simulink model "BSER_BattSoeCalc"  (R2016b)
settings: Solver=FixedStepDiscrete  StartTime=0.0  StopTime=10.0  FixedStep=0.02  RelTol=1e-3  EnableMultiTasking=on
undefined symbols (not defined in the file or in its folder): BSER_ahBattCapFilter_C, BSER_ahBattCapTemp_CUR, BSER_ahBattNrmCap_C, BSER_eBattSoeFilter_C, BSER_numSoeSeriesCells_C, BSER_rOCVSoc_A, BSER_rShrtPwrMapSoc_A, BSER_rSoeUsableRate_C, BSER_tBattCapTemp_A, BSER_tiSoeIniTime_C, BSER_uBattNrmVolt_C, BSER_uOCVSoc_CUR
libraries: simulink x4

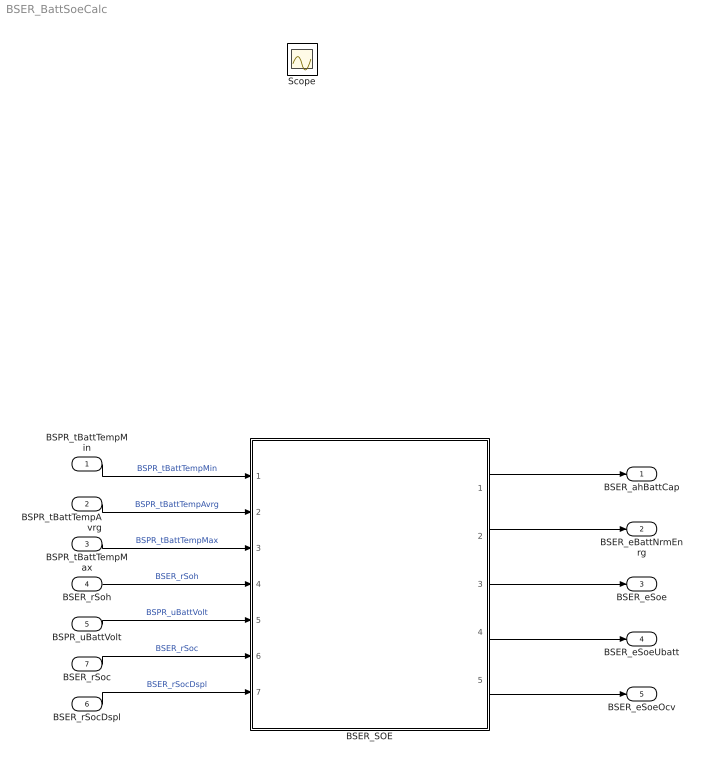
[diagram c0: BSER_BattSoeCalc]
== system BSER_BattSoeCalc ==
  BSPR_tBattTempMin : Inport
  BSPR_tBattTempAvrg : Inport  Port=2
  BSPR_tBattTempMax : Inport  Port=3
  BSER_rSoh : Inport  Port=4
  BSPR_uBattVolt : Inport  Port=5
  BSER_rSocDspl : Inport  Port=6
  BSER_rSoc : Inport  Port=7
  BSER_SOE : Subsystem  TreatAsAtomicUnit=on
  BSER_ahBattCap : Outport
  BSER_eBattNrmEnrg : Outport  Port=2
  BSER_eSoe : Outport  Port=3
  BSER_eSoeUbatt : Outport  Port=4
  BSER_eSoeOcv : Outport  Port=5
  Scope : Scope
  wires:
  BSPR_tBattTempAvrg/1 -> BSER_SOE/2(BSPR_tBattTempAvrg)  "BSPR_tBattTempAvrg"
  BSPR_tBattTempMin/1 -> BSER_SOE/1(BSPR_tBattTempMin)  "BSPR_tBattTempMin"
  BSPR_tBattTempMax/1 -> BSER_SOE/3(BSPR_tBattTempMax)  "BSPR_tBattTempMax"
  BSER_SOE/1(BSER_ahBattCap) -> BSER_ahBattCap/1
  BSER_rSoh/1 -> BSER_SOE/4(BSER_rSoh)  "BSER_rSoh"
  BSPR_uBattVolt/1 -> BSER_SOE/5(BSPR_uBattVolt)  "BSPR_uBattVolt"
  BSER_rSocDspl/1 -> BSER_SOE/7(BSER_rSocDspl)  "BSER_rSocDspl"
  BSER_SOE/2(BSER_eBattNrmEnrg) -> BSER_eBattNrmEnrg/1
  BSER_SOE/3(BSER_eSoe) -> BSER_eSoe/1
  BSER_SOE/4(BSER_eSoeUbatt) -> BSER_eSoeUbatt/1
  BSER_rSoc/1 -> BSER_SOE/6(BSER_rSoc)  "BSER_rSoc"
  BSER_SOE/5(BSER_eSoeOcv) -> BSER_eSoeOcv/1

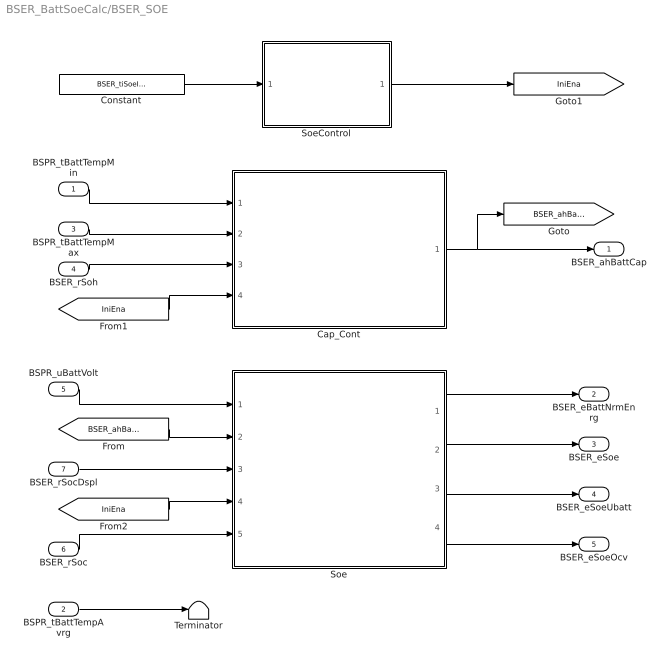
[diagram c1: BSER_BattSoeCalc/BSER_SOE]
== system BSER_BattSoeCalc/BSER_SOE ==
  BSPR_tBattTempMin : Inport
  BSPR_tBattTempAvrg : Inport  Port=2
  BSPR_tBattTempMax : Inport  Port=3
  BSER_rSoh : Inport  Port=4
  BSPR_uBattVolt : Inport  Port=5
  BSER_rSoc : Inport  Port=6
  BSER_rSocDspl : Inport  Port=7
  Cap_Cont : Subsystem  TreatAsAtomicUnit=on
  Constant : Constant  Value=BSER_tiSoeIniTime_C
  Soe : Subsystem
  SoeControl : Stateflow chart  TreatAsAtomicUnit=on
  Terminator : Terminator
  BSER_ahBattCap : Outport
  BSER_eBattNrmEnrg : Outport  Port=2
  BSER_eSoe : Outport  Port=3
  BSER_eSoeUbatt : Outport  Port=4
  BSER_eSoeOcv : Outport  Port=5
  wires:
  BSPR_tBattTempMin/1 -> Cap_Cont/1(BSPR_tBattTempMin)
  BSPR_tBattTempMax/1 -> Cap_Cont/2(BSPR_tBattTempMax)
  BSPR_tBattTempAvrg/1 -> Terminator/1
  Cap_Cont/1(BSER_ahBattCap) -> BSER_ahBattCap/1, [BSER_ahBattCap]
  BSER_rSoh/1 -> Cap_Cont/3(BSER_rSoh)
  BSPR_uBattVolt/1 -> Soe/1(BSPR_uBattVolt)
  BSER_rSocDspl/1 -> Soe/3(BSER_rSocDspl)
  Soe/1(BSER_eBattNrmEnrg) -> BSER_eBattNrmEnrg/1
  [BSER_ahBattCap] -> Soe/2(BSER_ahBattCap)
  Soe/2(BSER_eSoe) -> BSER_eSoe/1
  Soe/3(BSER_eSoeUbatt) -> BSER_eSoeUbatt/1
  Constant/1 -> SoeControl/1(IniTime)
  SoeControl/1(IniEna) -> [IniEna]
  [IniEna] -> Cap_Cont/4(IniEna)
  [IniEna] -> Soe/4(IniEna)
  BSER_rSoc/1 -> Soe/5(BSER_rSoc)
  Soe/4(BSER_eSoeOcv) -> BSER_eSoeOcv/1

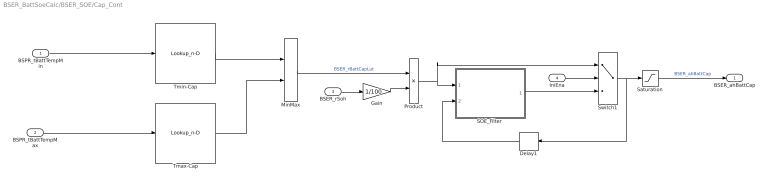
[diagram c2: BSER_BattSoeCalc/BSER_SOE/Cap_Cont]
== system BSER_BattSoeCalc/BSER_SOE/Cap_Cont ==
  BSPR_tBattTempMin : Inport
  BSPR_tBattTempMax : Inport  Port=2
  BSER_rSoh : Inport  Port=3
  IniEna : Inport  Port=4
  Delay1 : Delay  DelayLength=1  InitialCondition=0
  Gain : Gain  Gain=1/100
  MinMax : MinMax  Inputs=2  OutDataTypeStr=Inherit: Inherit via back propagation
  Product : Product  OutDataTypeStr=Inherit: Inherit via back propagation
  "SOE_Filter " : Subsystem
  Saturation : Saturate  UpperLimit=500  LowerLimit=1
  Switch1 : Switch  Criteria=u2 > Threshold
  Tmax-Cap : Lookup_n-D  NumberOfTableDimensions=1  BreakpointsForDimension1=BSER_tBattCapTemp_A  BreakpointsForDimension2=BSER_rShrtPwrMapSoc_A  Table=BSER_ahBattCapTemp_CUR  ExtrapMethod=Clip  UseLastTableValue=on  InternalRulePriority=Speed  RndMeth=Simplest
  Tmin-Cap : Lookup_n-D  NumberOfTableDimensions=1  BreakpointsForDimension1=BSER_tBattCapTemp_A  BreakpointsForDimension2=BSER_rShrtPwrMapSoc_A  Table=BSER_ahBattCapTemp_CUR  ExtrapMethod=Clip  UseLastTableValue=on  InternalRulePriority=Speed  RndMeth=Simplest
  BSER_ahBattCap : Outport
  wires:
  BSPR_tBattTempMin/1 -> Tmin-Cap/1
  BSPR_tBattTempMax/1 -> Tmax-Cap/1
  Tmin-Cap/1 -> MinMax/1
  Tmax-Cap/1 -> MinMax/2
  MinMax/1 -> Product/1  "BSER_rBattCapLut"
  BSER_rSoh/1 -> Gain/1
  Saturation/1 -> BSER_ahBattCap/1  "BSER_ahBattCap"
  Gain/1 -> Product/2
  Product/1 -> Switch1/1, "SOE_Filter "/1(CAPk)
  "SOE_Filter "/1(BSER_ahCap) -> Switch1/3
  Delay1/1 -> "SOE_Filter "/2(CAPk-1)
  Switch1/1 -> Delay1/1, Saturation/1
  IniEna/1 -> Switch1/2

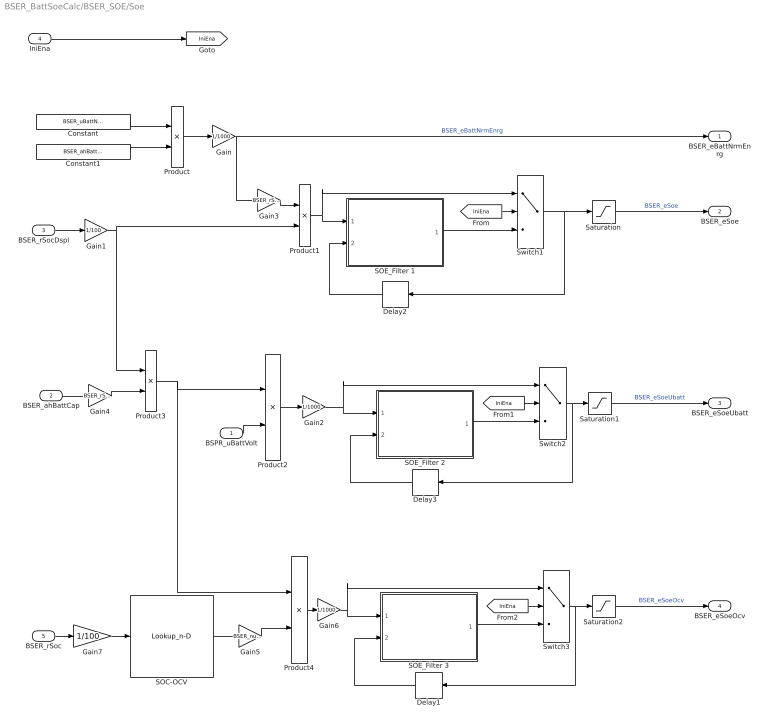
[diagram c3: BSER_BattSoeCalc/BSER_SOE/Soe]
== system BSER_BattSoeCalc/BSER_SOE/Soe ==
  BSPR_uBattVolt : Inport
  BSER_ahBattCap : Inport  Port=2
  BSER_rSocDspl : Inport  Port=3
  IniEna : Inport  Port=4
  BSER_rSoc : Inport  Port=5
  Constant : Constant  Value=BSER_uBattNrmVolt_C  SampleTime=-1
  Constant1 : Constant  Value=BSER_ahBattNrmCap_C  SampleTime=-1
  Delay1 : Delay  DelayLength=1  InitialCondition=0
  Delay2 : Delay  DelayLength=1  InitialCondition=0
  Delay3 : Delay  DelayLength=1  InitialCondition=0
  Gain : Gain  Gain=1/1000
  Gain1 : Gain  Gain=1/100
  Gain2 : Gain  Gain=1/1000
  Gain3 : Gain  Gain=BSER_rSoeUsableRate_C
  Gain4 : Gain  Gain=BSER_rSoeUsableRate_C
  Gain5 : Gain  Gain=BSER_numSoeSeriesCells_C
  Gain6 : Gain  Gain=1/1000
  Gain7 : Gain  Gain=1/100
  Product{,1..4} (5 alike) : Product  OutDataTypeStr=Inherit: Inherit via back propagation
  SOC-OCV : Lookup_n-D  NumberOfTableDimensions=1  BreakpointsForDimension1=BSER_rOCVSoc_A  BreakpointsForDimension2=BSER_rShrtPwrMapSoc_A  Table=BSER_uOCVSoc_CUR  ExtrapMethod=Clip  UseLastTableValue=on  InternalRulePriority=Speed  RndMeth=Simplest
  SOE_Filter 1 : Subsystem
  SOE_Filter 2 : Subsystem
  SOE_Filter 3 : Subsystem
  Saturation : Saturate  UpperLimit=500  LowerLimit=0
  Saturation1 : Saturate  UpperLimit=500  LowerLimit=0
  Saturation2 : Saturate  UpperLimit=500  LowerLimit=0
  Switch1 : Switch  Criteria=u2 > Threshold
  Switch2 : Switch  Criteria=u2 > Threshold
  Switch3 : Switch  Criteria=u2 > Threshold
  BSER_eBattNrmEnrg : Outport
  BSER_eSoe : Outport  Port=2
  BSER_eSoeUbatt : Outport  Port=3
  BSER_eSoeOcv : Outport  Port=4
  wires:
  BSER_rSocDspl/1 -> Gain1/1
  Constant1/1 -> Product/2
  Constant/1 -> Product/1
  Product/1 -> Gain/1
  Product3/1 -> Product4/1, Product2/1
  Product2/1 -> Gain2/1
  Gain/1 -> Gain3/1, BSER_eBattNrmEnrg/1  "BSER_eBattNrmEnrg"
  Gain1/1 -> Product1/2, Product3/1
  Saturation/1 -> BSER_eSoe/1  "BSER_eSoe"
  Product1/1 -> Switch1/1, SOE_Filter 1/1(SOEk)
  SOE_Filter 1/1(BSER_eSoe) -> Switch1/3
  Delay2/1 -> SOE_Filter 1/2(SOEk-1)
  Switch1/1 -> Delay2/1, Saturation/1
  [IniEna] -> Switch1/2
  Saturation1/1 -> BSER_eSoeUbatt/1  "BSER_eSoeUbatt"
  SOE_Filter 2/1(BSER_eSoe) -> Switch2/3
  Delay3/1 -> SOE_Filter 2/2(SoeRTk-1)
  Switch2/1 -> Delay3/1, Saturation1/1
  [IniEna] -> Switch2/2
  IniEna/1 -> [IniEna]
  Gain3/1 -> Product1/1
  Gain2/1 -> SOE_Filter 2/1(SoeRTk), Switch2/1
  BSER_ahBattCap/1 -> Gain4/1
  Gain4/1 -> Product3/2
  SOC-OCV/1 -> Gain5/1
  Gain5/1 -> Product4/2
  Gain7/1 -> SOC-OCV/1
  BSER_rSoc/1 -> Gain7/1
  Product4/1 -> Gain6/1
  Saturation2/1 -> BSER_eSoeOcv/1  "BSER_eSoeOcv"
  SOE_Filter 3/1(BSER_eSoe) -> Switch3/3
  Delay1/1 -> SOE_Filter 3/2(SoeRTk-1)
  Switch3/1 -> Delay1/1, Saturation2/1
  [IniEna] -> Switch3/2
  Gain6/1 -> SOE_Filter 3/1(SoeRTk), Switch3/1
  BSPR_uBattVolt/1 -> Product2/2

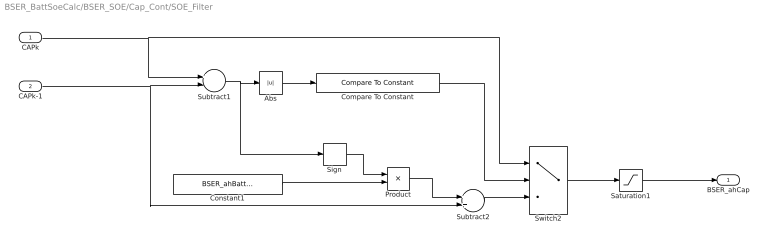
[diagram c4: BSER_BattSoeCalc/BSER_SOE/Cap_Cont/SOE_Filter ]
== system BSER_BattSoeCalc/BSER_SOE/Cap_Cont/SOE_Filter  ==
  CAPk : Inport
  CAPk-1 : Inport  Port=2
  Abs : Abs
  Compare To Constant : simulink/Logic and Bit Operations/Compare To Constant  relop=<=  const=BSER_ahBattCapFilter_C  OutDataTypeStr=boolean
  Constant1 : Constant  Value=BSER_ahBattCapFilter_C
  Product : Product
  Saturation1 : Saturate  UpperLimit=200  LowerLimit=0
  Sign : Signum
  Subtract1 : Sum  Inputs=+-
  Subtract2 : Sum
  Switch2 : Switch  Criteria=u2 > Threshold
  BSER_ahCap : Outport
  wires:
  CAPk-1/1 -> Subtract2/2, Subtract1/2
  Subtract1/1 -> Sign/1, Abs/1
  Abs/1 -> Compare To Constant/1
  Sign/1 -> Product/1
  Constant1/1 -> Product/2
  Product/1 -> Subtract2/1
  Subtract2/1 -> Switch2/3
  Compare To Constant/1 -> Switch2/2
  Saturation1/1 -> BSER_ahCap/1
  CAPk/1 -> Switch2/1, Subtract1/1
  Switch2/1 -> Saturation1/1

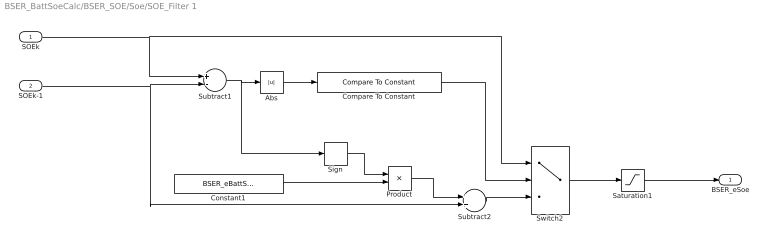
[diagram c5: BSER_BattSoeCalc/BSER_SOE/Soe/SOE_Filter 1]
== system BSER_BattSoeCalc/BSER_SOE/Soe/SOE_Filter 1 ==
  SOEk : Inport
  SOEk-1 : Inport  Port=2
  Abs : Abs
  Compare To Constant : simulink/Logic and Bit Operations/Compare To Constant  relop=<=  const=BSER_eBattSoeFilter_C  OutDataTypeStr=boolean
  Constant1 : Constant  Value=BSER_eBattSoeFilter_C  SampleTime=-1
  Product : Product
  Saturation1 : Saturate  UpperLimit=200  LowerLimit=0
  Sign : Signum
  Subtract1 : Sum  Inputs=+-
  Subtract2 : Sum
  Switch2 : Switch  Criteria=u2 > Threshold
  BSER_eSoe : Outport
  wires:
  SOEk-1/1 -> Subtract2/2, Subtract1/2
  Subtract1/1 -> Sign/1, Abs/1
  Abs/1 -> Compare To Constant/1
  Sign/1 -> Product/1
  Constant1/1 -> Product/2
  Product/1 -> Subtract2/1
  Subtract2/1 -> Switch2/3
  Compare To Constant/1 -> Switch2/2
  Saturation1/1 -> BSER_eSoe/1
  SOEk/1 -> Switch2/1, Subtract1/1
  Switch2/1 -> Saturation1/1

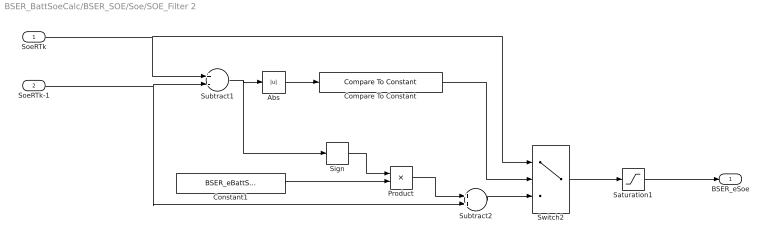
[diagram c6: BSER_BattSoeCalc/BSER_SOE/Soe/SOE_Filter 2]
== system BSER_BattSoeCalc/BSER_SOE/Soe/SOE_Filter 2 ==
  SoeRTk : Inport
  SoeRTk-1 : Inport  Port=2
  Abs : Abs
  Compare To Constant : simulink/Logic and Bit Operations/Compare To Constant  relop=<=  const=BSER_eBattSoeFilter_C  OutDataTypeStr=boolean
  Constant1 : Constant  Value=BSER_eBattSoeFilter_C  SampleTime=-1
  Product : Product
  Saturation1 : Saturate  UpperLimit=200  LowerLimit=0
  Sign : Signum
  Subtract1 : Sum  Inputs=+-
  Subtract2 : Sum
  Switch2 : Switch  Criteria=u2 > Threshold
  BSER_eSoe : Outport
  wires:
  SoeRTk-1/1 -> Subtract2/2, Subtract1/2
  Subtract1/1 -> Sign/1, Abs/1
  Abs/1 -> Compare To Constant/1
  Sign/1 -> Product/1
  Constant1/1 -> Product/2
  Product/1 -> Subtract2/1
  Subtract2/1 -> Switch2/3
  Compare To Constant/1 -> Switch2/2
  Saturation1/1 -> BSER_eSoe/1
  SoeRTk/1 -> Switch2/1, Subtract1/1
  Switch2/1 -> Saturation1/1

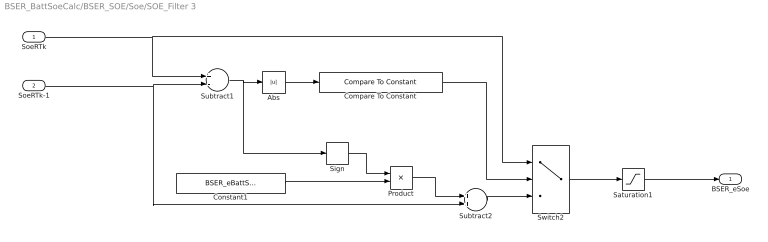
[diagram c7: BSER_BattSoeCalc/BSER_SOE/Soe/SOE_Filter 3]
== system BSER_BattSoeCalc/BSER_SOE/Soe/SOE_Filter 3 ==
  SoeRTk : Inport
  SoeRTk-1 : Inport  Port=2
  Abs : Abs
  Compare To Constant : simulink/Logic and Bit Operations/Compare To Constant  relop=<=  const=BSER_eBattSoeFilter_C  OutDataTypeStr=boolean
  Constant1 : Constant  Value=BSER_eBattSoeFilter_C  SampleTime=-1
  Product : Product
  Saturation1 : Saturate  UpperLimit=200  LowerLimit=0
  Sign : Signum
  Subtract1 : Sum  Inputs=+-
  Subtract2 : Sum
  Switch2 : Switch  Criteria=u2 > Threshold
  BSER_eSoe : Outport
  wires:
  Switch2/1 -> Saturation1/1
  SoeRTk/1 -> Subtract1/1, Switch2/1
  Saturation1/1 -> BSER_eSoe/1
  Compare To Constant/1 -> Switch2/2
  Subtract2/1 -> Switch2/3
  Product/1 -> Subtract2/1
  Constant1/1 -> Product/2
  Sign/1 -> Product/1
  Abs/1 -> Compare To Constant/1
  Subtract1/1 -> Abs/1, Sign/1
  SoeRTk-1/1 -> Subtract1/2, Subtract2/2

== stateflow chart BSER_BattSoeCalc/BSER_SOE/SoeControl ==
  state Ini
    entry:
    IniEna=logical(1);
  state Run
    entry:
    IniEna=logical(0);
  (default) -> Ini
  Ini -> Run : [after(IniTime,sec)]
  data: IniTime input; IniEna output
